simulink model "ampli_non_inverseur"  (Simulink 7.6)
settings: Solver=ode15s  StartTime=0.0  StopTime=N  RelTol=1e-3
InitFcn:
  | N=0.3;
  | Ad=10^5;
  | Vsat=15;
StopFcn:
  | close all, clc
  | load  ES_ampli_non_inverseur.mat
  | plot(x(1,:),x(2,:))
  | hold on
  | plot(x(1,:),x(3,:))
  | axis([0 N -20 20])
  | grid
  | title('Tension de sortie et d''entrée - Montage non inverseur')
  | xlabel('temps')
libraries: fl_lib x24, nesl_utility x4

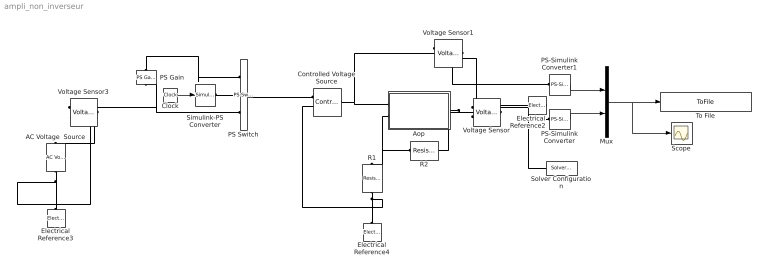
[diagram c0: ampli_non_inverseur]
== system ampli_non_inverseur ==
  AC Voltage  Source : fl_lib/Electrical/Electrical Sources/AC Voltage Source  DialogController=NetworkEngine.DynNeDlgSource  SystemSampleTime=-1  amp=7 V  shift=0 rad  omega=10 Hz  i_Log=off  v_Log=off  LocalVarNames=|current|voltage|power  LocalVarDescs=|Current (A)|Voltage (V)|Power (W)  LocalVarLogging=[0 0 0]
  Aop : Subsystem
  Clock : Clock
  Controlled Voltage Source : fl_lib/Electrical/Electrical Sources/Controlled Voltage Source  DialogController=NetworkEngine.DynNeDlgSource  SystemSampleTime=-1  i_Log=off  v_Log=off  LocalVarNames=|i|v  LocalVarDescs=|i|v  LocalVarLogging=[0 0]
  Electrical Reference2 : fl_lib/Electrical/Electrical Elements/Electrical Reference  DialogController=NetworkEngine.DynNeDlgSource  SystemSampleTime=-1  i_Log=off  LocalVarNames=|i  LocalVarDescs=|i  LocalVarLogging=[]
  Electrical Reference3 : fl_lib/Electrical/Electrical Elements/Electrical Reference  DialogController=NetworkEngine.DynNeDlgSource  SystemSampleTime=-1  i_Log=off  LocalVarNames=|i  LocalVarDescs=|i  LocalVarLogging=[]
  Electrical Reference4 : fl_lib/Electrical/Electrical Elements/Electrical Reference  DialogController=NetworkEngine.DynNeDlgSource  SystemSampleTime=-1  i_Log=off  LocalVarNames=|i  LocalVarDescs=|i  LocalVarLogging=[]
  Mux : Mux  Inputs=2
  PS Gain : fl_lib/Physical Signals/Functions/PS Gain  DialogController=NetworkEngine.DynNeDlgSource  SystemSampleTime=-1  gain=2  LocalVarLogging=[]
  PS Switch : fl_lib/Physical Signals/Nonlinear Operators/PS Switch  DialogController=NetworkEngine.DynNeDlgSource  SystemSampleTime=-1  Threshold=0.1  LocalVarLogging=[]
  PS-Simulink Converter : nesl_utility/PS-Simulink Converter  DialogController=NetworkEngine.DynNeUtilDlgSource  SystemSampleTime=-1  PhysicalDomain=network_engine_domain  LeftPortType=input  RightPortType=output  SubClassName=ps_output  Unit=1  AffineConversion=off
  PS-Simulink Converter1 : nesl_utility/PS-Simulink Converter  DialogController=NetworkEngine.DynNeUtilDlgSource  SystemSampleTime=-1  PhysicalDomain=network_engine_domain  LeftPortType=input  RightPortType=output  SubClassName=ps_output  Unit=1  AffineConversion=off
  R1 : fl_lib/Electrical/Electrical Elements/Resistor  DialogController=NetworkEngine.DynNeDlgSource  SystemSampleTime=-1  R=10 kOhm  i_Log=off  v_Log=off  LocalVarNames=|current|voltage|power  LocalVarDescs=|Resistor current (A)|Voltage across resistor (V)|Power (W)  LocalVarLogging=[0 0 0]
  R2 : fl_lib/Electrical/Electrical Elements/Resistor  DialogController=NetworkEngine.DynNeDlgSource  SystemSampleTime=-1  R=10 kOhm  i_Log=off  v_Log=off  LocalVarNames=|current|voltage|power  LocalVarDescs=|Resistor current (A)|Voltage across resistor (V)|Power (W)  LocalVarLogging=[0 0 0]
  Scope : Scope
  Simulink-PS Converter : nesl_utility/Simulink-PS Converter  DialogController=NetworkEngine.DynNeUtilDlgSource  SystemSampleTime=-1  PhysicalDomain=network_engine_domain  LeftPortType=input  RightPortType=output  SubClassName=ps_input  Unit=1  AffineConversion=off  InputFilterTimeConstant=.001  UdotUserProvided=0
  Solver Configuration : nesl_utility/Solver Configuration  DialogController=NetworkEngine.DynNeUtilDlgSource  SystemSampleTime=-1  PhysicalDomain=network_engine_domain  LeftPortType=input  RightPortType=generic  SubClassName=solver  Accelerate=off  Profile=off  ResidualTolerance=1e-9  MaxNonlinIter=12  MaxModeIter=2  DoFixedCost=off  UseLocalSampling=off  DoDC=off  LinearAlgebra=Sparse  LocalSolverSampleTime=.001  LocalSolverChoice=NE_BACKWARD_EULER_ADVANCER  UseLocalSolver=off
  To File : ToFile  Filename=ES_ampli_non_inverseur  MatrixName=x
  Voltage Sensor : fl_lib/Electrical/Electrical Sensors/Voltage Sensor  DialogController=NetworkEngine.DynNeDlgSource  SystemSampleTime=-1  i1_Log=off  v1_Log=off  LocalVarNames=|i1|v1  LocalVarDescs=|i1|v1  LocalVarLogging=[0 0]
  Voltage Sensor1 : fl_lib/Electrical/Electrical Sensors/Voltage Sensor  DialogController=NetworkEngine.DynNeDlgSource  SystemSampleTime=-1  i1_Log=off  v1_Log=off  LocalVarNames=|i1|v1  LocalVarDescs=|i1|v1  LocalVarLogging=[0 0]
  Voltage Sensor3 : fl_lib/Electrical/Electrical Sensors/Voltage Sensor  DialogController=NetworkEngine.DynNeDlgSource  SystemSampleTime=-1  i1_Log=off  v1_Log=off  LocalVarNames=|i1|v1  LocalVarDescs=|i1|v1  LocalVarLogging=[0 0]
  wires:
  PS-Simulink Converter1/1 -> Mux/1
  Mux/1 -> To File/1, Scope/1
  Clock/1 -> Simulink-PS Converter/1
  PS-Simulink Converter/1 -> Mux/2
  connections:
  AC Voltage  Source/RConn1 -- Electrical Reference3/LConn1 -- Voltage Sensor3/RConn2
  Aop/RConn1 -- Voltage Sensor/LConn1 -- R2/RConn1
  PS-Simulink Converter/LConn1 -- Voltage Sensor/RConn1 -- Solver Configuration/RConn1
  Voltage Sensor/RConn2 -- Electrical Reference2/LConn1 -- Voltage Sensor1/RConn2
  Aop/LConn2 -- R2/LConn1 -- R1/LConn1
  Voltage Sensor1/RConn1 -- PS-Simulink Converter1/LConn1
  R1/RConn1 -- Electrical Reference4/LConn1 -- Controlled Voltage Source/RConn2
  PS Switch/RConn1 -- Controlled Voltage Source/RConn1
  Controlled Voltage Source/LConn1 -- Aop/LConn1 -- Voltage Sensor1/LConn1
  Voltage Sensor3/LConn1 -- AC Voltage  Source/LConn1
  Simulink-PS Converter/RConn1 -- PS Switch/LConn2
  PS Switch/LConn3 -- Voltage Sensor3/RConn1 -- PS Gain/LConn1
  PS Gain/RConn1 -- PS Switch/LConn1

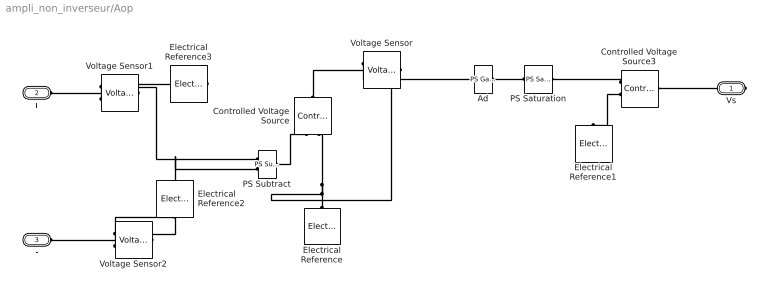
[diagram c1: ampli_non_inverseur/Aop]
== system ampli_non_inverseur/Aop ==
  Ad : fl_lib/Physical Signals/Functions/PS Gain  DialogController=NetworkEngine.DynNeDlgSource  SystemSampleTime=-1  gain=Ad  LocalVarLogging=[]
  Controlled Voltage Source : fl_lib/Electrical/Electrical Sources/Controlled Voltage Source  DialogController=NetworkEngine.DynNeDlgSource  SystemSampleTime=-1  i_Log=off  v_Log=off  LocalVarNames=|i|v  LocalVarDescs=|i|v  LocalVarLogging=[0 0]
  Controlled Voltage Source3 : fl_lib/Electrical/Electrical Sources/Controlled Voltage Source  DialogController=NetworkEngine.DynNeDlgSource  SystemSampleTime=-1  i_Log=off  v_Log=off  LocalVarNames=|i|v  LocalVarDescs=|i|v  LocalVarLogging=[0 0]
  Electrical Reference{,1..3} (4 alike) : fl_lib/Electrical/Electrical Elements/Electrical Reference  DialogController=NetworkEngine.DynNeDlgSource  SystemSampleTime=-1  i_Log=off  LocalVarNames=|i  LocalVarDescs=|i  LocalVarLogging=0
  PS Saturation : fl_lib/Physical Signals/Nonlinear Operators/PS Saturation  DialogController=NetworkEngine.DynNeDlgSource  SystemSampleTime=-1  upper_limit=Vsat  lower_limit=-Vsat  LocalVarLogging=[]
  PS Subtract : fl_lib/Physical Signals/Functions/PS Subtract  DialogController=NetworkEngine.DynNeDlgSource  SystemSampleTime=-1  LocalVarLogging=[]
  Voltage Sensor : fl_lib/Electrical/Electrical Sensors/Voltage Sensor  DialogController=NetworkEngine.DynNeDlgSource  SystemSampleTime=-1  i1_Log=off  v1_Log=off  LocalVarNames=|i1|v1  LocalVarDescs=|i1|v1  LocalVarLogging=[0 0]
  Voltage Sensor1 : fl_lib/Electrical/Electrical Sensors/Voltage Sensor  DialogController=NetworkEngine.DynNeDlgSource  SystemSampleTime=-1  i1_Log=off  v1_Log=off  LocalVarNames=|i1|v1  LocalVarDescs=|i1|v1  LocalVarLogging=[0 0]
  Voltage Sensor2 : fl_lib/Electrical/Electrical Sensors/Voltage Sensor  DialogController=NetworkEngine.DynNeDlgSource  SystemSampleTime=-1  i1_Log=off  v1_Log=off  LocalVarNames=|i1|v1  LocalVarDescs=|i1|v1  LocalVarLogging=[0 0]
  Vs : PMIOPort  Port=1  Side=Right
  + : PMIOPort  Port=2  Side=Left
  - : PMIOPort  Port=3  Side=Left
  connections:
  Voltage Sensor/RConn1 -- Ad/LConn1
  PS Saturation/LConn1 -- Ad/RConn1
  Controlled Voltage Source/LConn1 -- Voltage Sensor/LConn1
  PS Subtract/RConn1 -- Controlled Voltage Source/RConn1
  Electrical Reference/LConn1 -- Controlled Voltage Source/RConn2 -- Voltage Sensor/RConn2
  Controlled Voltage Source3/RConn1 -- PS Saturation/RConn1
  Controlled Voltage Source3/RConn2 -- Electrical Reference1/LConn1
  Vs/RConn1 -- Controlled Voltage Source3/LConn1
  +/RConn1 -- Voltage Sensor1/LConn1
  -/RConn1 -- Voltage Sensor2/LConn1
  Voltage Sensor2/RConn1 -- PS Subtract/LConn2
  Voltage Sensor1/RConn1 -- PS Subtract/LConn1
  Voltage Sensor1/RConn2 -- Electrical Reference3/LConn1
  Voltage Sensor2/RConn2 -- Electrical Reference2/LConn1
